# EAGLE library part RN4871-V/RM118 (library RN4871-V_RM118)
Bluetooth 4.2 BLE Module Shielded Antenna ASCII Interface 9x11.5mm
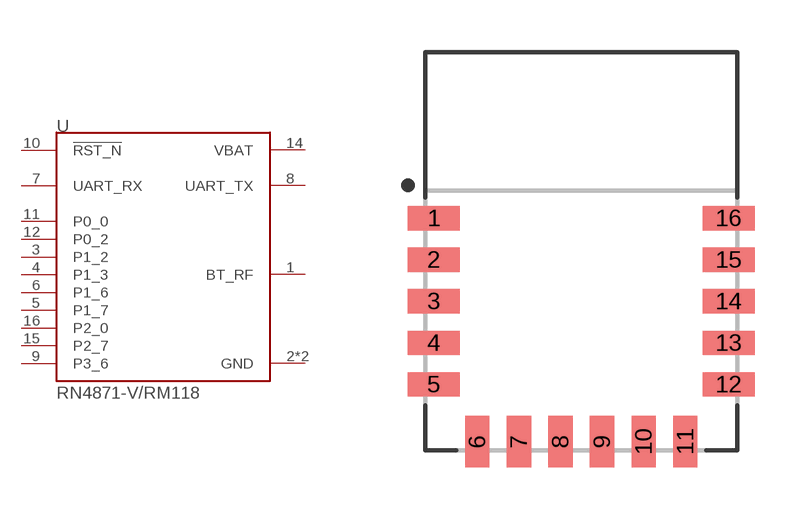
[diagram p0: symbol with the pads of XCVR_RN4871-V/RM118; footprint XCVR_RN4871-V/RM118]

Designator prefix U

## RN4871-V/RM118 (Availability: Good; Description: Bluetooth 4.2 BLE Module Shielded Antenna ASCII Interface 9x11.5mm; MF: Microchip; MP: RN4871-V/RM118; Package: SMD-16 Microchip; Price: 7.65 USD)  [XCVR_RN4871-V/RM118]
1  BT_RF
2  GND  pwr
3  P1_2
4  P1_3
5  P1_7
6  P1_6
7  UART_RX  in
8  UART_TX  out
9  P3_6
10  !RST_N  in
11  P0_0
12  P0_2
13  GND  pwr
14  VBAT  pwr
15  P2_7
16  P2_0

## Footprint XCVR_RN4871-V/RM118 (pad centres in mm)
smd 1.5 x 0.7: 1 -4.25,0.95; 2 -4.25,-0.25; 3 -4.25,-1.45; 4 -4.25,-2.65; 5 -4.25,-3.85; 12 4.25,-3.85; 13 4.25,-2.65; 14 4.25,-1.45; 15 4.25,-0.25; 16 4.25,0.95
smd 0.7 x 1.5: 6 -3,-5.5; 7 -1.8,-5.5; 8 -0.6,-5.5; 9 0.6,-5.5; 10 1.8,-5.5; 11 3,-5.5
